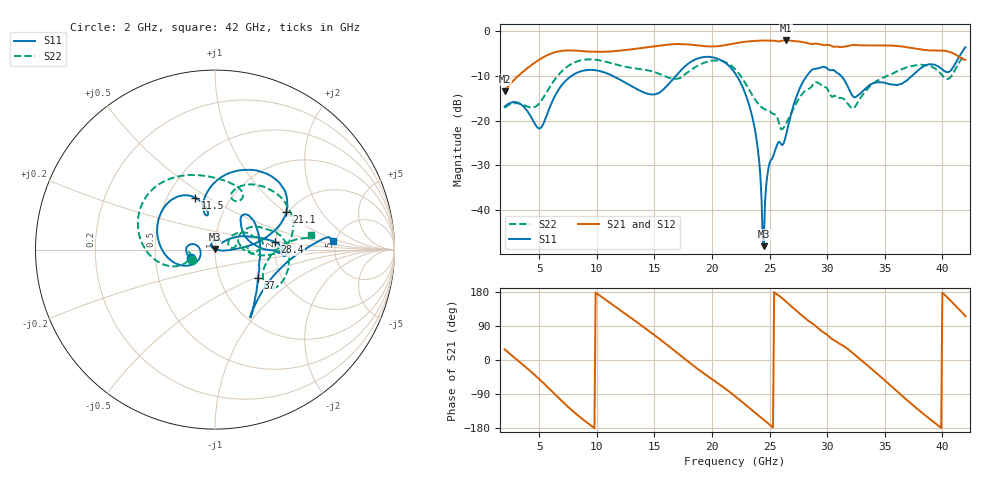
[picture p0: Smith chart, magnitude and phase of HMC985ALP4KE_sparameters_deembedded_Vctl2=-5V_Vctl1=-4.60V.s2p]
!s2p File: Measurements: S11, S21, S12, S22
# GHz S dB R 50.0
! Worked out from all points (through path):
!   401 points, 2 GHz to 42 GHz, reference 50 ohm
!   highest |S21| = -2.06 dB at 26.4 GHz (marker M1); lowest = -13.4 dB at 2 GHz (marker M2)
!   lowest |S11| = -48.1 dB at 24.5 GHz (marker M3), VSWR 1.01, Z = 49.8 + j0.301 ohm
!   |S11| at or under -10 dB: start of sweep to 7.807 GHz; 22.15 GHz to 28.23 GHz (6.082 GHz wide, 24.1 % of centre); 31.21 GHz to 37.36 GHz (6.155 GHz wide, 18 % of centre)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
!   |S22| runs from -22.0 to -5.3 dB; largest |S21 - S12| = 0.00097
!   S11 on the Smith chart (normalised r, x): 2 GHz: 0.76, -0.07; 11.5 GHz: 0.68, +0.44; 21.1 GHz: 1.97, +1.02; 28.4 GHz: 2.00, +0.19; 37 GHz: 1.52, -0.52; 42 GHz: 4.74, +0.85
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2  -16.87 -161.7  -13.43 28.3  -13.44 28.3  -17.17 -155.6
5  -21.78 -172.4  -6.38 -50.1  -6.38 -50.1  -16.18 -159.8
6.3  -14.84 -150.3  -4.76 -88.3  -4.76 -88.3  -11.04 -161.5
8.7  -8.90 150.4  -4.44 -154.5  -4.44 -154.5  -6.47 151.3
11.5  -10.16 111.1  -4.47 143.2  -4.47 143.2  -7.32 105.2
13.6  -13.11 101.2  -3.85 97.2  -3.85 97.2  -8.42 75.8
15.4  -13.81 105.8  -3.26 56.5  -3.25 56.5  -9.51 62.3
17.9  -7.33 80.3  -2.94 -3.4  -2.95 -3.4  -9.19 72.2
21.1  -6.97 27.6  -3.14 -74.3  -3.14 -74.2  -6.87 16.2
22  -9.37 17.0  -2.71 -95.5  -2.71 -95.4  -8.46 0.7
23.6  -20.32 -0.1  -2.18 -135.2  -2.18 -135.1  -14.73 -4.1
24.5  -48.14 129.5  -2.08 -157.8  -2.08 -157.8  -17.37 8.3
25  -29.53 133.3  -2.11 -170.6  -2.11 -170.5  -17.92 10.9
26.4  -23.57 42.3  -2.06 154.8  -2.06 154.8  -20.82 33.2
28.4  -9.43 7.2  -2.73 102.8  -2.73 102.8  -12.89 18.6
28.7  -8.61 2.2  -2.86 96.6  -2.87 96.6  -12.20 16.7
30.7  -8.96 -2.9  -3.45 50.9  -3.45 50.9  -14.49 2.6
32.5  -14.69 32.5  -3.09 11.0  -3.08 11.0  -16.60 28.1
35.4  -11.80 19.2  -3.18 -64.5  -3.18 -64.4  -9.81 19.5
37  -10.84 -33.3  -3.61 -107.6  -3.60 -107.5  -8.02 5.2
39.8  -8.16 -57.0  -4.32 -177.0  -4.32 -176.9  -9.33 -35.1
42  -3.60 4.4  -6.37 115.4  -6.37 115.5  -5.34 8.9
